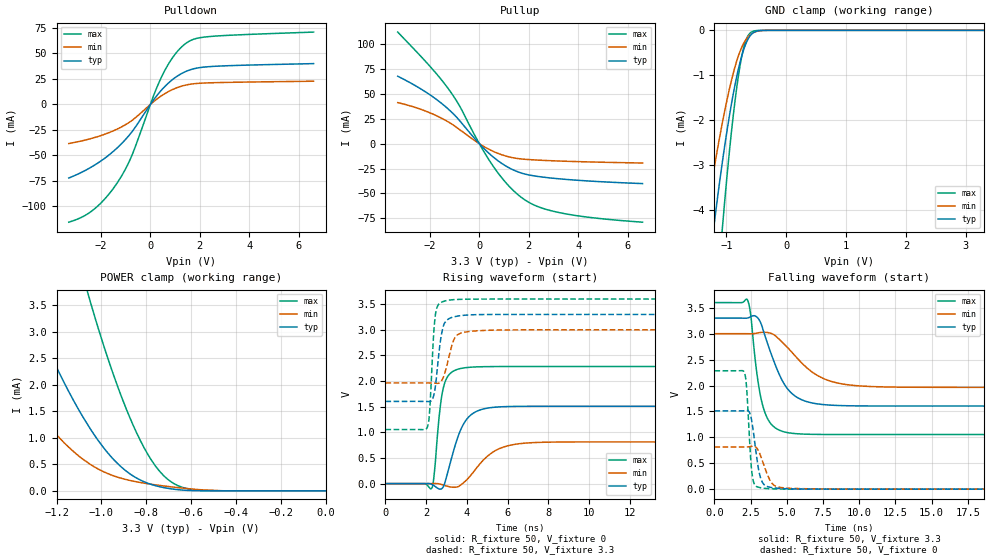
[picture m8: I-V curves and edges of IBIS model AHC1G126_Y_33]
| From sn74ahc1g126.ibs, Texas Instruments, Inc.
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[Model]   AHC1G126_Y_33
Model_type  3-state
Enable   Active-High
Vref =   0
Rref =   1000
Cref =   50p
Vmeas =   1.65
| variable   typ   min   max
C_comp   2.80pF   2.37pF   3.01pF
| C_pullup   4.06pF   2.53pF   5.07pF
| C_pulldown   5.20pF   3.09pF   8.71pF
| C_tri-state   2.80pF   2.37pF   3.01pF
[Temperature Range]   40   100   -40
| Ambient temperature   25   85   -40
[Voltage range]   3.3   3   3.6
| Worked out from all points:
|   slope of the pulldown table from 0 to 0.495 V, typ, clamps not added: 32.3 ohm
|   slope of the pullup table from 0 to 0.495 V, typ, clamps not added: 41.2 ohm
|   GND clamp passes 1 mA (typ) near -0.82 V on its own axis
|   POWER clamp passes 1 mA (typ) near -1.02 V on its own axis
|   rising waveform, R_fixture 50, V_fixture 0: 20-80 % time 793ps typ, 1.24ns min, 363ps max; typ from 0 V to 1.51 V
|   falling waveform, R_fixture 50, V_fixture 3.3: 20-80 % time 1.54ns typ, 2.42ns min, 782ps max; typ from 3.3 V to 1.6 V
|   rising waveform, R_fixture 50, V_fixture 3.3: 20-80 % time 310ps typ, 421ps min, 207ps max; typ from 1.6 V to 3.3 V
|   falling waveform, R_fixture 50, V_fixture 0: 20-80 % time 470ps typ, 676ps min, 286ps max; typ from 1.51 V to 0 V
[GND Clamp]
| AHC1G126_Y_33
|   Voltage   I(typ)   I(min)   I(max)
-3.3V     -41.29mA   -27.62mA   -63.42mA
-1.365V   -6.183mA   -4.403mA   -9.863mA
-1.35V    -6mA       -4.273mA   -9.556mA
-1.2V     -4.277mA   -3.039mA   -6.665mA
-1.065V   -2.914mA   -2.046mA   -4.374mA
-905mV    -1.561mA   -1.059mA   -2.131mA
-785mV    -781.4uA   -515.6uA   -891.6uA
-735mV    -531.9uA   -353.2uA   -522.8uA
-675mV    -299.9uA   -209.3uA   -225.4uA
-560mV    -61.62uA   -59.85uA   -23.23uA
-305mV    -378nA     -548.6nA   -22.17nA
3.3V      168pA      26.63nA    3.503pA
[POWER Clamp]
| AHC1G126_Y_33
|   Voltage   I(typ)   I(min)   I(max)
-3.3V     39.15mA    24.34mA    67.14mA
-1.615V   6.939mA    3.73mA     14.64mA
-1.365V   3.941mA    1.959mA    9.109mA
-1.325V   3.522mA    1.718mA    8.31mA
-1.085V   1.412mA    605.2uA    4.092mA
-1.05V    1.172mA    501.4uA    3.571mA
-945mV    589.1uA    283.5uA    2.172mA
-845mV    246.5uA    172.8uA    1.111mA
-780mV    125uA      126.8uA    598.2uA
-700mV    46.04uA    82.19uA    203.1uA
-550mV    1.827uA    19.73uA    9.061uA
-48.03fV  168pA      645.8pA    4.332pA
[Pulldown]
| AHC1G126_Y_33
|   Voltage   I(typ)   I(min)   I(max)
-3.3V     -72.15mA   -38.32mA   -115.4mA
-2.265V   -59.6mA    -32.52mA   -102.5mA
-1.77V    -51.36mA   -28.53mA   -90.63mA
-1.305V   -41.74mA   -23.7mA    -75.59mA
-750mV    -26.94mA   -15.77mA   -50.13mA
120mV     4.149mA    2.514mA    7.997mA
470mV     14.65mA    8.839mA    27.88mA
925mV     24.94mA    14.91mA    46.81mA
1.4V      31.98mA    18.83mA    59.28mA
1.78V     35.14mA    20.36mA    64.17mA
2.36V     37.04mA    21.18mA    66.52mA
6.6V      40.04mA    22.78mA    70.95mA
[Pullup]
| AHC1G126_Y_33
|   Voltage   I(typ)   I(min)   I(max)
-3.3V     67.9mA     41.34mA    112.3mA
-2.18V    52.21mA    32.88mA    82.93mA
-1.305V   35.91mA    22.62mA    57mA
-825mV    23.98mA    14.68mA    39.11mA
-30mV     818.4uA    489.4uA    1.343mA
500mV     -12.13mA   -7.016mA   -20.44mA
1.085V    -22.65mA   -12.52mA   -39.58mA
1.665V    -29.25mA   -15.28mA   -53.39mA
2.315V    -32.78mA   -16.45mA   -62.81mA
3.23V     -35.36mA   -17.44mA   -69.34mA
4.61V     -37.83mA   -18.45mA   -74.61mA
6.6V      -40.16mA   -19.46mA   -79.01mA
[Ramp]
| AHC1G126_Y_33
| variable   typ   min   max
dV/dt_r   0.97/8.17E-10   0.53/1.30E-09   1.43/3.81E-10
dV/dt_f   1.05/1.56E-09   0.64/2.46E-09   1.57/7.87E-10
R_load = 50
[Rising Waveform]
| AHC1G126_Y_33
R_fixture =   50
C_fixture =   0
L_fixture =   0
V_fixture =   0
V_fixture_min = 0
V_fixture_max = 0
|   Time   V(typ)   V(min)   V(max)
0s        123.8pV    220pV      53.87pV
2.28ns    -15.77mV   842.7uV    -85.11mV
2.39ns    -41.36mV   1.41mV     164.3mV
2.68ns    -108.4mV   -8.6mV     1.455V
2.86ns    -50.48mV   -28.81mV   1.891V
3.735ns   1.083V     -15.02mV   2.249V
4.315ns   1.373V     222.2mV    2.274V
5.28ns    1.487V     614.7mV    2.283V
6.89ns    1.508V     790.6mV    2.284V
29.99ns   1.51V      813.7mV    2.284V
[Falling Waveform]
| AHC1G126_Y_33
R_fixture =   50
C_fixture =   0
L_fixture =   0
V_fixture =   3.3
V_fixture_min = 3
V_fixture_max = 3.6
|   Time   V(typ)   V(min)   V(max)
0s        3.3V       3V         3.6V
2.28ns    3.302V     2.999V     3.651V
2.505ns   3.327V     2.998V     3.362V
2.99ns    3.304V     3.014V     2.115V
3.325ns   3.106V     3.026V     1.623V
3.865ns   2.651V     3.01V      1.273V
4.725ns   2.075V     2.824V     1.113V
6.195ns   1.706V     2.389V     1.062V
9.3ns     1.609V     2.011V     1.054V
29.99ns   1.604V     1.964V     1.054V
[Rising Waveform]
| AHC1G126_Y_33
R_fixture =   50
C_fixture =   0
L_fixture =   0
V_fixture =   3.3
V_fixture_min = 3
V_fixture_max = 3.6
|   Time   V(typ)   V(min)   V(max)
0s        1.604V     1.964V     1.054V
2.05ns    1.602V     1.964V     1.094V
2.165ns   1.601V     1.964V     1.384V
2.355ns   1.695V     1.961V     2.832V
2.465ns   1.936V     1.958V     3.325V
2.745ns   2.892V     1.998V     3.537V
3.01ns    3.184V     2.29V      3.571V
3.48ns    3.263V     2.883V     3.591V
4.545ns   3.296V     2.982V     3.599V
29.99ns   3.3V       3V         3.6V
[Falling Waveform]
| AHC1G126_Y_33
R_fixture =   50
C_fixture =   0
L_fixture =   0
V_fixture =   0
V_fixture_min = 0
V_fixture_max = 0
|   Time   V(typ)   V(min)   V(max)
0s        1.51V      813.7mV    2.284V
2.08ns    1.513V     813.1mV    2.241V
2.225ns   1.519V     814.1mV    1.939V
2.5ns     1.416V     822.6mV    596.8mV
2.59ns    1.293V     827.6mV    315mV
3.025ns   421.4mV    748.3mV    38.84mV
3.345ns   116.9mV    518.7mV    20.26mV
3.92ns    32.4mV     132.1mV    7.561mV
4.82ns    10.58mV    24.31mV    1.85mV
29.99ns   124.2pV    1.649nV    53.84pV
